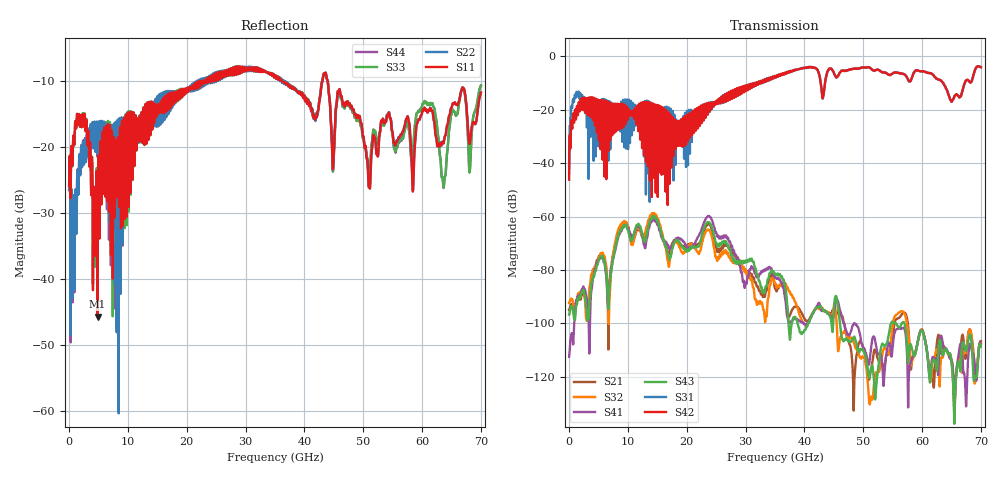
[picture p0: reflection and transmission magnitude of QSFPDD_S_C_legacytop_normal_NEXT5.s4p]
! AWR Design Environment (8415) Thu Dec 20 13:56:47 2018
! Document = 'CHANNEL TEST'
! nPorts: 4, nXvals: 7001
# HZ S DB R 50
!Freq DBS11 AngS11 DBS12 AngS12 DBS13 AngS13 DBS14 AngS14
!	DBS21 AngS21 DBS22 AngS22 DBS23 AngS23 DBS24 AngS24
!	DBS31 AngS31 DBS32 AngS32 DBS33 AngS33 DBS34 AngS34
!	DBS41 AngS41 DBS42 AngS42 DBS43 AngS43 DBS44 AngS44
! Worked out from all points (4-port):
!   7000 points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, 10 MHz to 70 GHz, reference 50 ohm
!   strongest paths, dB at 10 MHz, 17.51 GHz, 35.01 GHz, 52.51 GHz, 70 GHz:
!     S42: -46.2, -26.2, -7.4, -5.0, -4.0
!     S31: -42.3, -24.0, -7.5, -5.0, -4.0
!     S43: -96.7, -72.3, -81.6, -117.3, -108.6
!     S41: -112.5, -70.8, -82.9, -111.3, -107.7
!     S32: -92.3, -71.7, -85.1, -118.2, -107.5
!     S21: -94.9, -70.0, -86.9, -113.3, -106.6
!   lowest |S11| = -45.7 dB at 4.85 GHz (marker M1), VSWR 1.01, Z = 49.9 + j0.506 ohm
!   |S11| at or under -10 dB: start of sweep to 22.11 GHz; 36.16 GHz to 43.05 GHz (6.896 GHz wide, 17.4 % of centre); 43.97 GHz to end of sweep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
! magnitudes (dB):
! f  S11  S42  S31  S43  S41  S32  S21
! 10 MHz  -25.9  -46.2  -42.3  -96.7  -112.5  -92.3  -94.9
! 1.28 GHz  -16.1  -19.4  -13.3  -93.0  -91.4  -91.1  -91.9
! 4.85 GHz  -45.7  -16.7  -20.5  -78.0  -77.1  -76.9  -76.2
! 14.38 GHz  -14.2  -30.4  -32.2  -60.1  -61.2  -58.8  -59.6
! 16.95 GHz  -13.1  -21.4  -19.1  -75.7  -71.7  -78.7  -74.0
! 63.65 GHz  -19.4  -10.2  -10.2  -111.3  -109.2  -111.4  -108.6
! 70 GHz  -11.8  -4.0  -4.0  -108.6  -107.7  -107.5  -106.6
